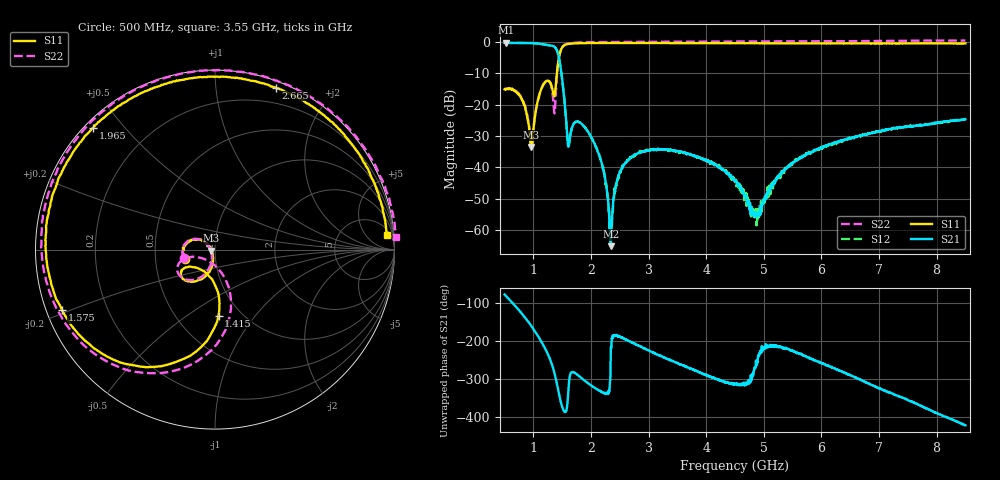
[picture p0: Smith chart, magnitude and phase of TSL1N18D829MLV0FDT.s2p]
! TSL1N18D829MLV0FDT  S-PARAMETER MODEL  ( General Type )
! Model Generated by TAIYO YUDEN Corporation (https://www.yuden.co.jp/en/)
! Version 1.0
! TAIYO YUDEN Control No. 20130917
! Copyright(c) 2013 TAIYO YUDEN CO.,LTD. All Rights Reserved.
! Products Name : Multilayer Ceramic Devices
! Characteristics :
!  Passband freq : 698-960MHz ( At Passband , Insertion Loss : 0.45dB , VSWR 2.0 ),
!  Attenuation : 15dB min at 1554-1610MHz) , 21dB min at 1760-1830MHz , Impedance : 50 Ohm ,
!  Case Size : 1.6 x 0.8 / 0.063 x 0.031 [mm/inch] , Thickness : 0.65 / 0.026 [mm/inch]
!  (Conditions: Temperature = 25 degC , DC Bias Current/Voltage = 0A / 0V)
! External Node Assignments :
!  1  o---|-------|---o  2
!  |  LPF  |
! GND o---|-------|---o GND
! Frequency Range : 500MHz  -  8.5GHz  [ 1601 STEP ]
# MHZ S RI R 50
! Freq[MHz].  S11 Real  S11 Imag  S21 Real  S21 Imag  S12 Real  S12 Imag  S22 Real  S22 Imag
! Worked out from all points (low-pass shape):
!   1601 points, 500 MHz to 8.5 GHz, reference 50 ohm
!   highest |S21| = -0.26 dB at 520 MHz (marker M1); lowest = -65.1 dB at 2.345 GHz (marker M2)
!   |S21| within 3 dB of the highest: start of sweep to 1.419 GHz
!   lowest |S11| = -33.5 dB at 965 MHz (marker M3), VSWR 1.04, Z = 48 - j0.542 ohm
!   |S11| at or under -10 dB: start of sweep to 1.408 GHz
!   |S22| runs from -32.5 to 0.5 dB; largest |S21 - S12| = 0.0041
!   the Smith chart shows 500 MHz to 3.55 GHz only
!   S11 on the Smith chart (normalised r, x): 500 MHz: 0.71, -0.08; 1.415 GHz: 0.79, -0.67; 1.575 GHz: 0.05, -0.19; 1.965 GHz: 0.02, +0.41; 2.665 GHz: 0.06, +1.44; 3.55 GHz: 10, +19
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500  -0.1676 -0.0541  0.2191 -0.9451  0.2178 -0.9456  -0.1719 -0.0493
520  -0.169 -0.0424  0.1661 -0.9566  0.1662 -0.956  -0.1754 -0.0405
795  -0.1086 0.0588  -0.5718 -0.7747  -0.5727 -0.7743  -0.1134 0.0595
965  -0.0204 -0.00565  -0.905 -0.3269  -0.9036 -0.3242  -0.0229 -0.00627
1120  -0.0562 -0.1517  -0.8933 0.2697  -0.8945 0.2702  -0.0704 -0.148
1290  -0.1886 -0.1241  -0.3227 0.8207  -0.3246 0.8198  -0.2062 -0.0874
1360  -0.0742 -0.1139  0.1599 0.8295  0.1585 0.8307  -0.0577 -0.0532
1415  0.02 -0.3681  0.5228 0.4746  0.5243 0.4735  0.0891 -0.3263
1575  -0.8526 -0.3365  0.0428 -0.0169  0.0427 -0.0166  -0.8515 -0.3834
1835  -0.8426 0.4552  0.0231 0.044  0.0231 0.0436  -0.8702 0.4597
1965  -0.678 0.6797  0.0239 0.0255  0.0241 0.0257  -0.7039 0.6989
2200  -0.3274 0.9054  0.00937 0.00415  0.00914 0.00407  -0.3354 0.9373
2345  -0.1061 0.9579  -0.000451 0.00032  -0.000523 0.00082  -0.1055 0.994
2470  0.0753 0.9605  -0.007 0.00107  -0.007 0.000979  0.088 0.9961
2665  0.3402 0.9023  -0.0129 0.00475  -0.0125 0.00476  0.3614 0.9338
3170  0.82 0.5019  -0.0106 0.0163  -0.0108 0.0158  0.8663 0.5142
3550  0.9567 0.0791  -0.00239 0.0175  -0.00264 0.017  1.007 0.0692
4500  0.4834 -0.8242  0.00424 0.00447  0.00384 0.0044  0.5021 -0.887
4890  0.0645 -0.9519  -0.000357 0.00166  -0.00068 0.00185  0.0567 -1.021
5835  -0.8288 -0.4635  -0.00678 0.0163  -0.00718 0.0159  -0.8997 -0.4937
7170  -0.4428 0.836  0.0371 0.0162  0.0371 0.0168  -0.4987 0.9139
8500  0.8159 0.48  0.0268 -0.0518  0.0278 -0.0522  0.9 0.5479
